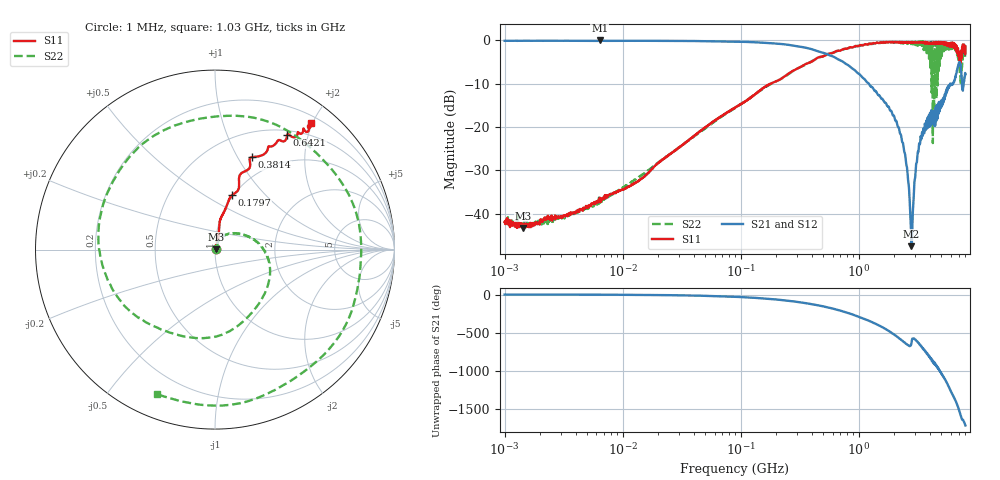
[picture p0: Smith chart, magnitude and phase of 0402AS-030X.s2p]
!s-Parameter Generated by FASTRON Sdn. Bhd.
!FASTRON P/N : 0402AS-030X
!Keysight Technologies: E5071C_MY46733604_B.14.02
!Date: Mon Dec 01 10:34:10 2025
!Version  :Rev00  Mon Dec 01 10:34:10 2025
!Data & Calibration Information:
!Freq  S11:SOLT2(ON)  S21:SOLT2(ON)  S12:SOLT2(ON)  S22:SOLT2(ON)
!PortZ  Port1:50+j0  Port2:50+j0
!When reading reference impedance value at option line is always used.
! Remarks : This data is being provided solely for informational purposes.
# Hz S dB R 50
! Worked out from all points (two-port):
!   1601 points, 1 MHz to 8 GHz, reference 50 ohm
!   highest |S21| = 0.00 dB at 6.4 MHz (marker M1); lowest = -47.5 dB at 2.795 GHz (marker M2)
!   |S21| within 3 dB of the highest: start of sweep to 519.2 MHz
!   lowest |S11| = -43.3 dB at 1.441 MHz (marker M3), VSWR 1.01, Z = 50.6 + j0.254 ohm
!   |S11| at or under -10 dB: start of sweep to 178.5 MHz
!   |S22| runs from -43.1 to -0.1 dB; largest |S21 - S12| = 0.01
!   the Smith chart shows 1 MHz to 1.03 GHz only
!   S11 on the Smith chart (normalised r, x): 1 MHz: 1.02, +0.01; 179.7 MHz: 0.99, +0.67; 381.4 MHz: 0.77, +1.15; 642.1 MHz: 0.57, +1.67; 1.03 GHz: 0.30, +1.97
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1000000  -41.90 21.8  -0.08 -0.4  -0.06 -0.3  -41.70 15.6
1441002  -43.30 21.5  -0.07 -0.5  -0.06 -0.5  -42.40 9.2
4479405  -39.00 49.5  -0.08 -1.6  -0.07 -1.5  -39.40 51.7
6400096  -36.30 57.6  0.00 -2.3  -0.02 -2.0  -36.70 50.4
2.00676e7  -28.30 71.7  -0.09 -6.8  -0.09 -6.7  -28.10 68.6
8.994653e7  -15.50 80.1  -0.26 -29.8  -0.25 -29.8  -15.50 31.2
1.796504e8  -9.96 72.6  -0.64 -58.4  -0.63 -58.4  -10.10 -14.9
3.814186e8  -5.12 68.2  -1.87 -121.0  -1.86 -121.0  -5.12 -132.0
4.006501e8  -4.88 65.5  -2.03 -127.0  -2.01 -127.0  -4.77 -141.0
6.42063e8  -2.46 57.8  -4.07 164.0  -4.06 164.0  -2.59 89.3
1.030344e9  -1.06 52.9  -7.98 61.6  -7.98 61.5  -1.23 -112.0
1.349549e9  -0.65 57.5  -11.50 -14.7  -11.50 -14.7  -0.66 89.6
1.550632e9  -0.51 62.6  -13.40 -60.2  -13.40 -60.3  -0.46 -6.8
1.7949e9  -0.36 68.3  -15.30 -117.0  -15.40 -117.0  -0.51 -126.0
2.061212e9  -0.47 73.5  -18.60 -179.0  -18.60 -179.0  -0.40 105.0
2.252141e9  -0.55 76.1  -21.60 136.0  -21.60 136.0  -0.40 10.9
2.472225e9  -0.48 80.9  -26.40 85.6  -26.40 85.6  -0.75 -102.0
2.795014e9  -0.38 89.8  -47.50 84.1  -47.30 84.8  -0.58 98.4
3.183204e9  -0.38 99.2  -25.80 88.9  -25.80 88.7  -0.71 -96.3
3.548043e9  -0.41 110.0  -20.50 -1.8  -20.50 -2.2  -2.21 71.4
3.892614e9  -0.65 116.0  -19.50 -70.1  -19.50 -70.6  -0.41 -77.2
8e9  -1.36 -110.0  -7.79 88.0  -7.76 87.6  -3.32 130.0
